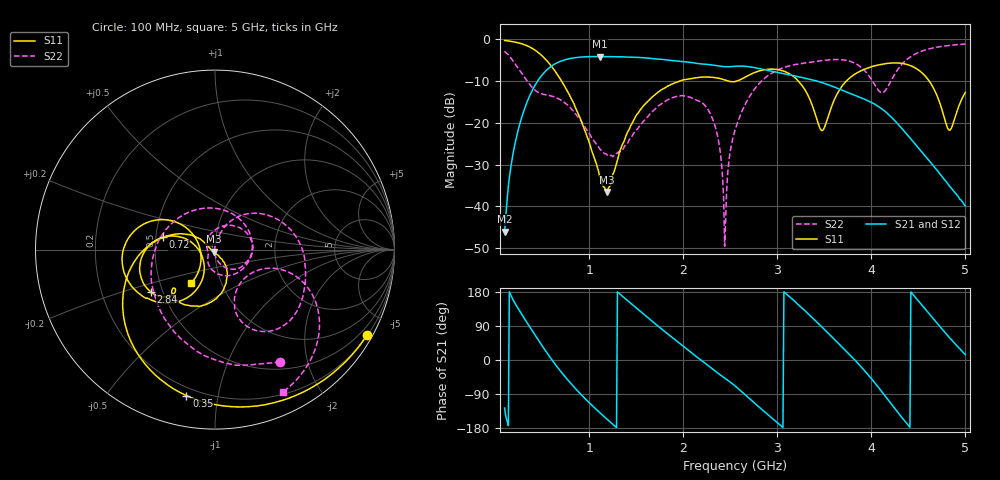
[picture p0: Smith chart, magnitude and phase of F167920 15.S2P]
!  2-Port S-parameters saved by WinCal
! VAR MeasName=S-Parameters (CALIBRATED_DATA) read from VNA (N5242A)
! VAR MeasDate=2016-11-22 9:54:19
! VAR NAME=F167920 15
! VAR FILENAME=F167920 15.S2P
! VAR DATE=2016-11-22 9:54:19
! VAR PHYS_PORTS=1,2
# Hz S DB R 50
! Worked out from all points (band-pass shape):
!   491 points, 100 MHz to 5 GHz, reference 50 ohm
!   highest |S21| = -4.10 dB at 1.11 GHz (marker M1); lowest = -46.1 dB at 100 MHz (marker M2)
!   |S21| within 3 dB of the highest: 559.4 MHz to 2.835 GHz (2.275 GHz wide, 134 % of centre)
!   lowest |S11| = -36.6 dB at 1.19 GHz (marker M3), VSWR 1.03, Z = 49.2 - j1.22 ohm
!   |S11| at or under -10 dB: 706.5 MHz to 1.962 GHz (1.256 GHz wide, 94.1 % of centre); 3.224 GHz to 3.734 GHz (509.6 MHz wide, 14.6 % of centre); 4.615 GHz to end of sweep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
!   |S22| runs from -49.6 to -1.1 dB; largest |S21 - S12| = 0.0019
!   S11 on the Smith chart (normalised r, x): 100 MHz: 0.22, -3.82; 350 MHz: 0.16, -0.81; 720 MHz: 0.55, +0.08; 2.84 GHz: 0.43, -0.25; 5 GHz: 0.71, -0.28
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1e8  -0.25 -29.3  -46.06 -126.7  -45.81 -126.1  -2.81 -59.8
2e8  -0.59 -57.9  -26.16 154.2  -26.15 154.3  -5.49 -110.9
3.5e8  -1.63 -101.1  -14.39 94.0  -14.39 94.0  -10.28 164.6
5.1e8  -4.18 -146.1  -8.22 33.4  -8.21 33.4  -13.14 57.6
7.2e8  -10.50 166.8  -5.04 -37.2  -5.03 -37.2  -14.84 -44.6
9.2e8  -19.84 144.1  -4.21 -92.8  -4.20 -92.8  -19.75 -106.7
1.11e9  -32.73 175.4  -4.10 -138.5  -4.10 -138.5  -26.18 -141.9
1.19e9  -36.61 -122.8  -4.11 -156.4  -4.11 -156.4  -27.67 -156.1
1.46e9  -19.90 -55.7  -4.27 145.7  -4.27 145.7  -23.01 125.6
1.74e9  -12.52 -80.0  -4.73 87.8  -4.72 87.8  -15.87 57.5
2.26e9  -9.04 -126.6  -6.00 -13.9  -5.98 -13.9  -16.74 -48.8
2.38e9  -9.32 -134.5  -6.37 -36.9  -6.37 -36.9  -25.04 -79.4
2.44e9  -9.71 -136.9  -6.53 -47.6  -6.52 -47.7  -49.57 -133.0
2.55e9  -10.09 -134.7  -6.44 -68.1  -6.43 -68.2  -21.75 74.0
2.84e9  -7.37 -146.5  -7.13 -131.5  -7.10 -131.6  -9.81 38.4
3.37e9  -15.72 160.2  -9.68 112.2  -9.67 112.1  -5.40 -20.9
3.48e9  -21.85 -153.5  -10.40 85.7  -10.39 85.6  -5.07 -29.5
3.74e9  -9.85 -121.3  -12.64 21.4  -12.63 21.4  -5.06 -53.1
4.19e9  -5.70 -162.4  -18.14 -109.2  -18.14 -109.5  -10.71 -21.5
4.57e9  -8.72 153.3  -27.88 135.4  -27.91 135.0  -2.55 -39.1
4.83e9  -21.79 -171.7  -35.14 59.3  -35.14 58.7  -1.44 -56.0
5e9  -12.68 -125.7  -39.87 14.6  -39.89 13.6  -1.11 -64.6
